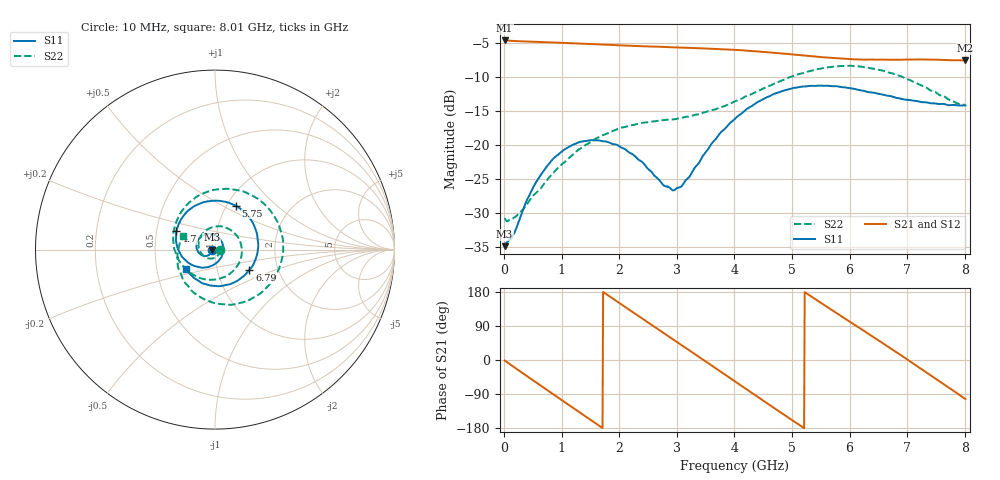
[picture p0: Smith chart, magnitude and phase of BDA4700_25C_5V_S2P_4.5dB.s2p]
!Agilent Technologies,E5071B,MY42404982,A.09.10
!Date: Mon Oct 20 13:28:09 2025
!Data & Calibration Information:
!Freq	S11:SOLT2(ON)	S21:SOLT2(ON)	S12:SOLT2(ON)	S22:SOLT2(ON)
# Hz S RI R 50
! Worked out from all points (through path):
!   801 points, 10 MHz to 8.01 GHz, reference 50 ohm
!   highest |S21| = -4.62 dB at 10 MHz (marker M1); lowest = -7.6 dB at 8.01 GHz (marker M2)
!   group delay of S21, straight-line fit = 284 ps
!   lowest |S11| = -34.9 dB at 10 MHz (marker M3), VSWR 1.04, Z = 48.2 - j0.119 ohm
!   |S11| at or under -10 dB: start of sweep to end of sweep
!   |S22| runs from -31.3 to -8.3 dB; largest |S21 - S12| = 0.0046
!   S11 on the Smith chart (normalised r, x): 10 MHz: 0.96, -0.00; 4.7 GHz: 0.63, +0.14; 5.75 GHz: 1.10, +0.58; 6.79 GHz: 1.43, -0.34; 8.01 GHz: 0.71, -0.16
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1e7  -0.0179 -0.00124  0.5873 -0.0124  0.5875 -0.0133  0.0287 -0.00252
3.3e8  -0.0249 -0.022  0.4721 -0.3343  0.4719 -0.3345  0.0205 -0.0263
7.2e8  -0.0571 -0.0354  0.1348 -0.5541  0.1348 -0.5542  -0.0181 -0.05
1.02e9  -0.0883 -0.0199  -0.1711 -0.5371  -0.1716 -0.5371  -0.0637 -0.0351
1.35e9  -0.1038 0.0196  -0.4388 -0.3419  -0.4394 -0.3418  -0.0919 0.0258
1.93e9  -0.0555 0.084  -0.502 0.2055  -0.5024 0.206  0.00235 0.1284
2.32e9  0.00188 0.0784  -0.2473 0.4738  -0.2471 0.4737  0.1101 0.0906
2.68e9  0.0399 0.039  0.086 0.5212  0.0866 0.5207  0.1494 -0.018
2.96e9  0.0457 -0.0076  0.3229 0.4108  0.3229 0.41  0.1143 -0.1037
3.36e9  0.0123 -0.0703  0.5065 0.0954  0.507 0.0951  -0.00363 -0.1673
3.67e9  -0.048 -0.0985  0.4737 -0.1846  0.4736 -0.1859  -0.1099 -0.1459
4.01e9  -0.1309 -0.084  0.2765 -0.4174  0.2766 -0.4172  -0.1989 -0.0631
4.35e9  -0.1994 -0.0122  -0.0142 -0.489  -0.0144 -0.4901  -0.2333 0.0672
4.7e9  -0.2153 0.1025  -0.2918 -0.3757  -0.2912 -0.3766  -0.1851 0.2145
5.35e9  -0.0467 0.2678  -0.436 0.1085  -0.4366 0.1077  0.1186 0.3322
5.75e9  0.1155 0.2446  -0.2565 0.352  -0.2559 0.3521  0.3138 0.2096
6.19e9  0.2278 0.1083  0.0539 0.4211  0.0576 0.4215  0.3735 -0.0479
6.68e9  0.2154 -0.0794  0.352 0.2355  0.353 0.2351  0.2039 -0.2734
6.79e9  0.1917 -0.1134  0.3905 0.1642  0.3914 0.1622  0.146 -0.2958
7.31e9  0.0334 -0.2031  0.367 -0.2147  0.367 -0.2153  -0.1205 -0.2386
7.67e9  -0.0816 -0.1809  0.1608 -0.3891  0.16 -0.3902  -0.2076 -0.0817
8.01e9  -0.1609 -0.1107  -0.0943 -0.4075  -0.0941 -0.4078  -0.181 0.0768
